| TEXAS INSTRUMENTS INCORPORATED
| Standard Linear and Logic Group
| IBIS Model of SN74CB3Q16245
| 16-bit Switch 2.5-V/3.3-V Low Voltage FET Bus Switch
| This file contains package information for the following:
|  TSSOP 48-pin (DGG) package as [Component] CB3Q16245_DGG
|  TVSOP 48-pin (DGV) package as [Component] CB3Q16245_DGV
|  SSOP 48-pin (DL) package as [Component] CB3Q16245_DL
| This device can be powered at the following Vccs:
|  3.3 volt Vcc
|  2.5 volt Vcc
| This file provides unique models under the [Model Selector] for each Vcc.
| For operation at a specific Vcc, select the appropriate model after each
| [Model Selector] keyword.
[IBIS Ver]   3.2
[Comment char]  |_char
[File Name]   sn74cb3q16245.ibs
[File Rev]   1.1 | x_die
[Date]   August 23, 2004
[Source]   Data created from TI-SPICE simulations at TI-SLL.
[Notes]   The following is an IBIS list for the CB3Q16245.
   Please contact sllibis@ti.com with questions and
   comments concerning SLL IBIS models.
   - FILE REV HISTORY
   - 1.1 Release IBIS file on 10/18/04
   - Power clamp data deleted as there is no power-clamp diode.
[Disclaimer] Property of Texas Instruments Incorporated.  Unauthorized
   reproduction and/or distribution is strictly prohibited.
   This product is protected under copyright law.
   Created  2003, (C) Copyright  2003, Texas Instruments
   Incorporated, All Rights Reserved
   UNLESS THERE IS A SIGNED, WRITTEN AGREEMENT TO THE
   CONTRARY, TEXAS INSTRUMENTS (TI) IS PROVIDING THE IBIS
   MODELS  AND WITHOUT ANY WARRANTY, EXPRESSED OR
   IMPLIED.  TI assumes no liability for:
   1) the accuracy of the IBIS models provided to your
   company;
   2) the proper functioning of these IBIS Models in your
   design or for any resulting applications; or
   3) infringement of patents, copyrights or intellectual
   property rights resulting from your use of these IBIS
   models.
   TI provides IBIS Models as a service to our customers.
   You and your company shall not distribute, sell or give
   these models to anyone else without prior written
   permission from TI.
   TI reserves the right to make changes to our products or
   to discontinue any semiconductor product or service
   without notice, and advises our customers to obtain the
   latest version of relevant information to verify, before
   placing orders, that the information being relied on is
   current.
   Please be aware that your receipt and use of the IBIS
   information provided shall serve as acceptance of these
   terms and conditions.  If you do not accept these terms,
   you should return or destroy the IBIS models and any
   other accompanying information immediately.
| Component CB3Q16245_DGG 48-pin TSSOP
[Component]   CB3Q16245_DGG
[Manufacturer]   Texas Instruments, Inc.
[Package]
|   typ   min   max
R_pkg   6.200e-02   5.000e-02   7.800e-02
L_pkg   3.527e-09   3.128e-09   4.255e-09
C_pkg   5.300e-13   4.170e-13   6.850e-13
[Pin]   signal_name   model_name   R_pin   L_pin   C_pin
1   NC   NC   5.000e-02   4.250e-09   6.710e-13
2   1B1   CB3Q16245_IO   5.700e-02   3.956e-09   6.740e-13
3   1B2   CB3Q16245_IO   7.100e-02   3.922e-09   6.190e-13
4   GND   GND   7.800e-02   3.841e-09   6.180e-13
5   1B3   CB3Q16245_IO   5.600e-02   3.535e-09   5.550e-13
6   1B4   CB3Q16245_IO   5.800e-02   3.464e-09   5.030e-13
7   VCC   POWER   6.000e-02   3.362e-09   4.980e-13
8   1B5   CB3Q16245_IO   6.100e-02   3.293e-09   4.620e-13
9   1B6   CB3Q16245_IO   6.300e-02   3.240e-09   4.550e-13
10   GND   GND   6.300e-02   3.175e-09   4.420e-13
11   1B7   CB3Q16245_IO   6.400e-02   3.153e-09   4.290e-13
12   1B8   CB3Q16245_IO   6.500e-02   3.128e-09   4.180e-13
13   2B1   CB3Q16245_IO   6.500e-02   3.128e-09   4.180e-13
14   2B2   CB3Q16245_IO   6.400e-02   3.154e-09   4.290e-13
15   GND   GND   6.300e-02   3.174e-09   4.420e-13
16   2B3   CB3Q16245_IO   6.300e-02   3.241e-09   4.550e-13
17   2B4   CB3Q16245_IO   6.100e-02   3.293e-09   4.620e-13
18   VCC   POWER   6.000e-02   3.362e-09   4.970e-13
19   2B5   CB3Q16245_IO   5.800e-02   3.464e-09   5.030e-13
20   2B6   CB3Q16245_IO   5.600e-02   3.537e-09   5.600e-13
21   GND   GND   7.700e-02   3.839e-09   6.260e-13
22   2B7   CB3Q16245_IO   7.100e-02   3.917e-09   6.270e-13
23   2B8   CB3Q16245_IO   5.800e-02   3.955e-09   6.850e-13
24   NC   NC   5.200e-02   4.255e-09   6.790e-13
25   2NOE   CB3Q16245_IN   5.100e-02   4.254e-09   6.760e-13
26   2A8   CB3Q16245_IO   5.800e-02   3.957e-09   6.790e-13
27   2A7   CB3Q16245_IO   7.100e-02   3.920e-09   6.210e-13
28   GND   GND   7.800e-02   3.843e-09   6.220e-13
29   2A6   CB3Q16245_IO   5.600e-02   3.539e-09   5.600e-13
30   2A5   CB3Q16245_IO   5.800e-02   3.466e-09   5.030e-13
31   VCC   POWER   6.000e-02   3.363e-09   4.970e-13
32   2A4   CB3Q16245_IO   6.100e-02   3.294e-09   4.620e-13
33   2A3   CB3Q16245_IO   6.300e-02   3.241e-09   4.540e-13
34   GND   GND   6.300e-02   3.175e-09   4.410e-13
35   2A2   CB3Q16245_IO   6.400e-02   3.153e-09   4.290e-13
36   2A1   CB3Q16245_IO   6.500e-02   3.129e-09   4.170e-13
37   1A8   CB3Q16245_IO   6.500e-02   3.129e-09   4.170e-13
38   1A7   CB3Q16245_IO   6.400e-02   3.152e-09   4.290e-13
39   GND   GND   6.400e-02   3.176e-09   4.410e-13
40   1A6   CB3Q16245_IO   6.300e-02   3.241e-09   4.540e-13
41   1A5   CB3Q16245_IO   6.100e-02   3.293e-09   4.620e-13
42   VCC   POWER   6.000e-02   3.363e-09   4.970e-13
43   1A4   CB3Q16245_IO   5.800e-02   3.464e-09   5.030e-13
44   1A3   CB3Q16245_IO   5.600e-02   3.534e-09   5.610e-13
45   GND   GND   7.800e-02   3.841e-09   6.260e-13
46   1A2   CB3Q16245_IO   7.100e-02   3.920e-09   6.220e-13
47   1A1   CB3Q16245_IO   5.700e-02   3.955e-09   6.770e-13
48   1NOE   CB3Q16245_IN   5.100e-02   4.252e-09   6.720e-13
| Component CB3Q16245_DGV 48-pin TVSOP
[Component]   CB3Q16245_DGV
[Manufacturer]   Texas Instruments, Inc.
[Package]
|   typ   min   max
R_pkg   7.000e-02   4.900e-02   8.500e-02
L_pkg   3.013e-09   2.743e-09   3.408e-09
C_pkg   3.710e-13   2.940e-13   5.110e-13
[Pin]   signal_name   model_name   R_pin   L_pin   C_pin
1   NC   NC   4.900e-02   3.393e-09   4.970e-13
2   1B1   CB3Q16245_IO   6.000e-02   3.250e-09   5.020e-13
3   1B2   CB3Q16245_IO   7.700e-02   3.310e-09   4.510e-13
4   GND   GND   8.500e-02   3.299e-09   4.040e-13
5   1B3   CB3Q16245_IO   8.300e-02   3.136e-09   3.600e-13
6   1B4   CB3Q16245_IO   7.700e-02   3.019e-09   3.630e-13
7   VCC   POWER   6.500e-02   2.882e-09   3.490e-13
8   1B5   CB3Q16245_IO   6.600e-02   2.829e-09   3.140e-13
9   1B6   CB3Q16245_IO   6.700e-02   2.796e-09   3.140e-13
10   GND   GND   6.900e-02   2.754e-09   3.080e-13
11   1B7   CB3Q16245_IO   7.000e-02   2.753e-09   3.010e-13
12   1B8   CB3Q16245_IO   7.100e-02   2.745e-09   2.940e-13
13   2B1   CB3Q16245_IO   7.000e-02   2.744e-09   2.940e-13
14   2B2   CB3Q16245_IO   7.000e-02   2.754e-09   3.010e-13
15   GND   GND   6.900e-02   2.754e-09   3.080e-13
16   2B3   CB3Q16245_IO   6.700e-02   2.796e-09   3.140e-13
17   2B4   CB3Q16245_IO   6.600e-02   2.829e-09   3.140e-13
18   VCC   POWER   6.500e-02   2.883e-09   3.500e-13
19   2B5   CB3Q16245_IO   7.500e-02   3.014e-09   3.630e-13
20   2B6   CB3Q16245_IO   8.000e-02   3.128e-09   3.580e-13
21   GND   GND   8.400e-02   3.295e-09   4.030e-13
22   2B7   CB3Q16245_IO   7.800e-02   3.311e-09   4.520e-13
23   2B8   CB3Q16245_IO   6.200e-02   3.259e-09   5.010e-13
24   NC   NC   5.200e-02   3.404e-09   4.960e-13
25   2NOE   CB3Q16245_IN   5.300e-02   3.397e-09   5.050e-13
26   2A8   CB3Q16245_IO   6.200e-02   3.249e-09   5.110e-13
27   2A7   CB3Q16245_IO   7.700e-02   3.308e-09   4.530e-13
28   GND   GND   8.200e-02   3.289e-09   4.030e-13
29   2A6   CB3Q16245_IO   7.800e-02   3.121e-09   3.590e-13
30   2A5   CB3Q16245_IO   7.400e-02   3.010e-09   3.630e-13
31   VCC   POWER   6.500e-02   2.883e-09   3.490e-13
32   2A4   CB3Q16245_IO   6.700e-02   2.829e-09   3.140e-13
33   2A3   CB3Q16245_IO   6.700e-02   2.795e-09   3.140e-13
34   GND   GND   6.900e-02   2.753e-09   3.070e-13
35   2A2   CB3Q16245_IO   7.000e-02   2.753e-09   3.010e-13
36   2A1   CB3Q16245_IO   7.000e-02   2.743e-09   2.940e-13
37   1A8   CB3Q16245_IO   7.000e-02   2.743e-09   2.940e-13
38   1A7   CB3Q16245_IO   7.000e-02   2.753e-09   3.010e-13
39   GND   GND   6.900e-02   2.754e-09   3.070e-13
40   1A6   CB3Q16245_IO   6.800e-02   2.797e-09   3.140e-13
41   1A5   CB3Q16245_IO   6.700e-02   2.830e-09   3.140e-13
42   VCC   POWER   6.400e-02   2.880e-09   3.490e-13
43   1A4   CB3Q16245_IO   7.200e-02   3.004e-09   3.620e-13
44   1A3   CB3Q16245_IO   7.800e-02   3.121e-09   3.590e-13
45   GND   GND   8.400e-02   3.296e-09   4.030e-13
46   1A2   CB3Q16245_IO   7.700e-02   3.308e-09   4.510e-13
47   1A1   CB3Q16245_IO   6.200e-02   3.258e-09   4.990e-13
48   1NOE   CB3Q16245_IN   5.300e-02   3.408e-09   4.940e-13
| Component CB3Q16245_DL 48-pin SSOP
[Component]   CB3Q16245_DL
[Manufacturer]   Texas Instruments, Inc.
[Package]
|   typ   min   max
R_pkg   4.800e-02   3.800e-02   5.300e-02
L_pkg   6.046e-09   5.084e-09   7.968e-09
C_pkg   8.130e-13   5.690e-13   1.157e-12
[Pin]   signal_name   model_name   R_pin   L_pin   C_pin
1   NC   NC   4.600e-02   7.968e-09   1.017e-12
2   1B1   CB3Q16245_IO   4.400e-02   7.299e-09   1.157e-12
3   1B2   CB3Q16245_IO   4.300e-02   6.765e-09   1.058e-12
4   GND   GND   4.100e-02   6.269e-09   9.330e-13
5   1B3   CB3Q16245_IO   3.800e-02   5.856e-09   8.290e-13
6   1B4   CB3Q16245_IO   4.600e-02   5.802e-09   7.900e-13
7   VCC   POWER   5.000e-02   5.656e-09   7.380e-13
8   1B5   CB3Q16245_IO   5.300e-02   5.500e-09   6.430e-13
9   1B6   CB3Q16245_IO   5.200e-02   5.304e-09   6.060e-13
10   GND   GND   5.300e-02   5.189e-09   5.830e-13
11   1B7   CB3Q16245_IO   5.100e-02   5.084e-09   5.690e-13
12   1B8   CB3Q16245_IO   5.300e-02   5.862e-09   8.330e-13
13   2B1   CB3Q16245_IO   5.300e-02   5.862e-09   8.330e-13
14   2B2   CB3Q16245_IO   5.100e-02   5.084e-09   5.690e-13
15   GND   GND   5.300e-02   5.189e-09   5.830e-13
16   2B3   CB3Q16245_IO   5.200e-02   5.304e-09   6.060e-13
17   2B4   GND   5.300e-02   5.500e-09   6.430e-13
18   VCC   POWER   5.000e-02   5.656e-09   7.380e-13
19   2B5   CB3Q16245_IO   4.600e-02   5.802e-09   7.900e-13
20   2B6   CB3Q16245_IO   3.800e-02   5.856e-09   8.290e-13
21   GND   GND   4.100e-02   6.269e-09   9.330e-13
22   2B7   CB3Q16245_IO   4.300e-02   6.765e-09   1.058e-12
23   2B8   CB3Q16245_IO   4.400e-02   7.299e-09   1.157e-12
24   NC   NC   4.600e-02   7.968e-09   1.017e-12
25   2NOE   CB3Q16245_IN   4.600e-02   7.968e-09   1.017e-12
26   2A8   CB3Q16245_IO   4.400e-02   7.299e-09   1.157e-12
27   2A7   CB3Q16245_IO   4.300e-02   6.765e-09   1.058e-12
28   GND   GND   4.100e-02   6.269e-09   9.330e-13
29   2A6   CB3Q16245_IO   3.800e-02   5.856e-09   8.290e-13
30   2A5   CB3Q16245_IO   4.600e-02   5.802e-09   7.900e-13
31   VCC   POWER   5.000e-02   5.656e-09   7.380e-13
32   2A4   CB3Q16245_IO   5.300e-02   5.500e-09   6.430e-13
33   2A3   CB3Q16245_IO   5.200e-02   5.304e-09   6.060e-13
34   GND   GND   5.300e-02   5.189e-09   5.830e-13
35   2A2   CB3Q16245_IO   5.100e-02   5.084e-09   5.690e-13
36   2A1   CB3Q16245_IO   5.300e-02   5.862e-09   8.330e-13
37   1A8   CB3Q16245_IO   5.300e-02   5.862e-09   8.330e-13
38   1A7   CB3Q16245_IO   5.100e-02   5.084e-09   5.690e-13
39   GND   GND   5.300e-02   5.189e-09   5.830e-13
40   1A6   CB3Q16245_IO   5.200e-02   5.304e-09   6.060e-13
41   1A5   CB3Q16245_IO   5.300e-02   5.500e-09   6.430e-13
42   VCC   POWER   5.000e-02   5.656e-09   7.380e-13
43   1A4   CB3Q16245_IO   4.600e-02   5.802e-09   7.900e-13
44   1A3   CB3Q16245_IO   3.800e-02   5.856e-09   8.290e-13
45   GND   GND   4.100e-02   6.269e-09   9.330e-13
46   1A2   CB3Q16245_IO   4.300e-02   6.765e-09   1.058e-12
47   1A1   CB3Q16245_IO   4.400e-02   7.299e-09   1.157e-12
48   1NOE   CB3Q16245_IN   4.600e-02   7.967e-09   1.017e-12
[Series Switch Groups]
| Function Group States
On  1 /   | 1A1-1A8->1B1-1B8 1NOE LOW
On  2 /   | 2A1-2A8->2B1-2B8 2NOE LOW
[Series Pin Mapping]   pin_2   model_name   function_table_group
37   12   CB3Q16245_IO_33_S   1
| 37   12   CB3Q16245_IO_25_S   1
38   11   CB3Q16245_IO_33_S   1
| 38   11   CB3Q16245_IO_25_S   1
40   9   CB3Q16245_IO_33_S   1
| 40   9   CB3Q16245_IO_25_S   1
41   8   CB3Q16245_IO_33_S   1
| 41   8   CB3Q16245_IO_25_S   1
43   6   CB3Q16245_IO_33_S   1
| 43   6   CB3Q16245_IO_25_S   1
44   5   CB3Q16245_IO_33_S   1
| 44   5   CB3Q16245_IO_25_S   1
46   3   CB3Q16245_IO_33_S   1
| 46   3   CB3Q16245_IO_25_S   1
47   2   CB3Q16245_IO_33_S   1
| 47   2   CB3Q16245_IO_25_S   1
26   23   CB3Q16245_IO_33_S   2
| 26   23   CB3Q16245_IO_25_S   2
27   22   CB3Q16245_IO_33_S   2
| 27   22   CB3Q16245_IO_25_S   2
29   20   CB3Q16245_IO_33_S   2
| 29   20   CB3Q16245_IO_25_S   2
30   19   CB3Q16245_IO_33_S   2
| 30   19   CB3Q16245_IO_25_S   2
32   17   CB3Q16245_IO_33_S   2
| 32   17   CB3Q16245_IO_25_S   2
33   16   CB3Q16245_IO_33_S   2
| 33   16   CB3Q16245_IO_25_S   2
35   14   CB3Q16245_IO_33_S   2
| 35   14   CB3Q16245_IO_25_S   2
36   13   CB3Q16245_IO_33_S   2
| 36   13   CB3Q16245_IO_25_S   2
| Model CB3Q16245_IN
[Model Selector]   CB3Q16245_IN
CB3Q16245_IN_33   3.3 volt Vcc
CB3Q16245_IN_25   2.5 volt Vcc
| Model CB3Q16245_IO
[Model Selector]   CB3Q16245_IO
CB3Q16245_IO_33   3.3 volt Vcc
CB3Q16245_IO_25   2.5 volt Vcc
| Model CB3Q16245_IO_S
[Model Selector]   CB3Q16245_IO_S
CB3Q16245_IO_33_S   3.3 volt Vcc
CB3Q16245_IO_25_S   2.5 volt Vcc
[Model]   CB3Q16245_IO_33_S
Model_type  Series_switch
| variable   typ   min   max
C_comp   0   0   0
[Temperature Range]   40   100   -40
| Ambient temperature   25   85   -40
[Voltage range]   3.3   3   3.6
[On]
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[Off]
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[Model]   CB3Q16245_IO_25_S
Model_type  Series_switch
| variable   typ   min   max
C_comp   0   0   0
[Temperature Range]   40   100   -40
| Ambient temperature   25   85   -40
[Voltage range]   2.5   2.3   2.7
[On]
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[Off]
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| Models and submodels in the file (6): CB3Q16245_IN_33 (Input), CB3Q16245_IN_25 (Input), CB3Q16245_IO_33_S (Series_switch), CB3Q16245_IO_33 (Terminator), CB3Q16245_IO_25_S (Series_switch), CB3Q16245_IO_25 (Terminator)
